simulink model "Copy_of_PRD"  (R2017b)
settings: Solver=FixedStepDiscrete  StartTime=0.0  StopTime=10.0  FixedStep=0.01  RelTol=1e-3  EnableMultiTasking=on
undefined symbols (not defined in the file): CcPRD_MaxPreChrgCnt_numb, CcPRD_PackCurrRat_pct, CcPRD_PreChrgCrntRvsCrntThrd_A, CcPRD_PreChrgCrntRvsDebTi_ms, CcPRD_PreChrgFailWaitTi_s, CcPRD_PreChrgR_ohm, CcPRD_PreChrgShrtDebTi_ms, CcPRD_PreChrgVoltRat_pct, CcPRD_VoltDiff_V, Enum_CTCCtrCtlState, PRD_CONST0_NUMB, PRD_CONST165_NUMB, PRD_CONST60_NUMB, PRD_RUNTIME_MS
libraries: AIWAYS_Powertrain_BMS_lib x17

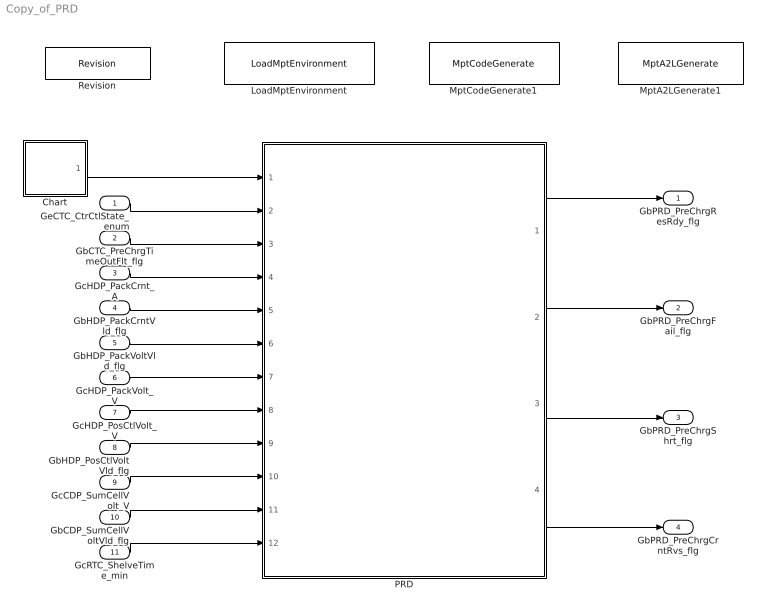
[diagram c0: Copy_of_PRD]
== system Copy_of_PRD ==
  GeCTC_CtrCtlState_enum : Inport
  GbCTC_PreChrgTimeOutFlt_flg : Inport  Port=2
  GcHDP_PackCrnt_A : Inport  Port=3
  GbHDP_PackCrntVld_flg : Inport  Port=4
  GbHDP_PackVoltVld_flg : Inport  Port=5
  GcHDP_PackVolt_V : Inport  Port=6
  GcHDP_PosCtlVolt_V : Inport  Port=7
  GbHDP_PosCtlVoltVld_flg : Inport  Port=8
  GcCDP_SumCellVolt_V : Inport  Port=9
  GbCDP_SumCellVoltVld_flg : Inport  Port=10
  GcRTC_ShelveTime_min : Inport  Port=11
  Chart : Stateflow chart  TreatAsAtomicUnit=on
  LoadMptEnvironment : AIWAYS_Powertrain_BMS_lib/Config/LoadMptEnvironment  ProjectName=Comm  SuppierID=NewPlatformUAES
  MptA2LGenerate1 : AIWAYS_Powertrain_BMS_lib/Config/MptA2LGenerate  SystemSampleTime=-1
  MptCodeGenerate1 : AIWAYS_Powertrain_BMS_lib/Config/MptCodeGenerate  SystemSampleTime=-1
  PRD : Subsystem
  Revision : AIWAYS_Powertrain_BMS_lib/Config/Revision  curVersion='M100C100R101'  newVersion='M100C100R101'
  GbPRD_PreChrgResRdy_flg : Outport
  GbPRD_PreChrgFail_flg : Outport  Port=2
  GbPRD_PreChrgShrt_flg : Outport  Port=3
  GbPRD_PreChrgCrntRvs_flg : Outport  Port=4
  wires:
  GcHDP_PackCrnt_A/1 -> PRD/4(GcHDP_PackCrnt_A)
  GbCTC_PreChrgTimeOutFlt_flg/1 -> PRD/3(GbCTC_PreChrgTimeOutFlt_flg)
  GbHDP_PackCrntVld_flg/1 -> PRD/5(GbHDP_PackCrntVld_flg)
  GeCTC_CtrCtlState_enum/1 -> PRD/2(GeCTC_CtrCtlState_enum)
  GbHDP_PackVoltVld_flg/1 -> PRD/6(GbHDP_PackVoltVld_flg)
  GcHDP_PackVolt_V/1 -> PRD/7(GcHDP_PackVolt_V)
  GcHDP_PosCtlVolt_V/1 -> PRD/8(GcHDP_PosCtlVolt_V)
  GbHDP_PosCtlVoltVld_flg/1 -> PRD/9(GbHDP_PosCtlVoltVld_flg)
  GcCDP_SumCellVolt_V/1 -> PRD/10(GcCDP_SumCellVolt_V)
  GbCDP_SumCellVoltVld_flg/1 -> PRD/11(GbCDP_SumCellVoltVld_flg)
  GcRTC_ShelveTime_min/1 -> PRD/12(GcRTC_ShelveTime_min)
  PRD/1(GbPRD_PreChrgResRdy_flg) -> GbPRD_PreChrgResRdy_flg/1
  PRD/2(GbPRD_PreChrgFail_flg) -> GbPRD_PreChrgFail_flg/1
  PRD/3(GbPRD_PreChrgShrt_flg) -> GbPRD_PreChrgShrt_flg/1
  PRD/4(GbPRD_PreChrgCrntRvs_flg) -> GbPRD_PreChrgCrntRvs_flg/1
  Chart/1(PRD_PreChrgResDiag_10ms()) -> PRD/1(PRD_PreChrgResDiag_10ms)

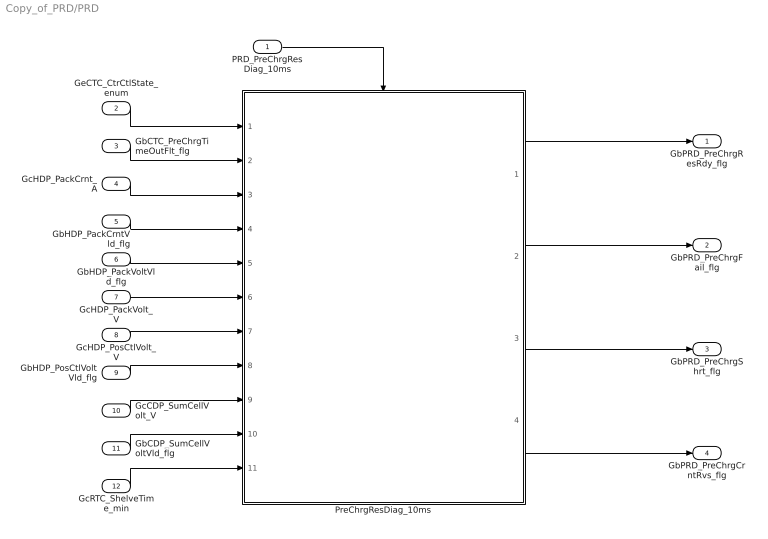
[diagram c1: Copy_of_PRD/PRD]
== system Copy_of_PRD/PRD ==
  PRD_PreChrgResDiag_10ms : Inport
  GeCTC_CtrCtlState_enum : Inport  Port=2
  GbCTC_PreChrgTimeOutFlt_flg : Inport  Port=3
  GcHDP_PackCrnt_A : Inport  Port=4
  GbHDP_PackCrntVld_flg : Inport  Port=5
  GbHDP_PackVoltVld_flg : Inport  Port=6
  GcHDP_PackVolt_V : Inport  Port=7
  GcHDP_PosCtlVolt_V : Inport  Port=8
  GbHDP_PosCtlVoltVld_flg : Inport  Port=9
  GcCDP_SumCellVolt_V : Inport  Port=10
  GbCDP_SumCellVoltVld_flg : Inport  Port=11
  GcRTC_ShelveTime_min : Inport  Port=12
  PreChrgResDiag_10ms : Subsystem
  GbPRD_PreChrgResRdy_flg : Outport
  GbPRD_PreChrgFail_flg : Outport  Port=2
  GbPRD_PreChrgShrt_flg : Outport  Port=3
  GbPRD_PreChrgCrntRvs_flg : Outport  Port=4
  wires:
  GeCTC_CtrCtlState_enum/1 -> PreChrgResDiag_10ms/1(GeCTC_CtrCtlState_enum)
  GbCTC_PreChrgTimeOutFlt_flg/1 -> PreChrgResDiag_10ms/2(GbCTC_PreChrgTimeOutFlt_flg)
  GcHDP_PackCrnt_A/1 -> PreChrgResDiag_10ms/3(GcHDP_PackCrnt_A)
  GbHDP_PackCrntVld_flg/1 -> PreChrgResDiag_10ms/4(GbHDP_PackCrntVld_flg)
  GbHDP_PackVoltVld_flg/1 -> PreChrgResDiag_10ms/5(GbHDP_PackVoltVld_flg)
  GcHDP_PackVolt_V/1 -> PreChrgResDiag_10ms/6(GcHDP_PackVolt_V)
  GcHDP_PosCtlVolt_V/1 -> PreChrgResDiag_10ms/7(GcHDP_PosCtlVolt_V)
  GbHDP_PosCtlVoltVld_flg/1 -> PreChrgResDiag_10ms/8(GbHDP_PosCtlVoltVld_flg)
  GcCDP_SumCellVolt_V/1 -> PreChrgResDiag_10ms/9(GcCDP_SumCellVolt_V)
  GbCDP_SumCellVoltVld_flg/1 -> PreChrgResDiag_10ms/10(GbCDP_SumCellVoltVld_flg)
  GcRTC_ShelveTime_min/1 -> PreChrgResDiag_10ms/11(GcRTC_ShelveTime_min)
  PreChrgResDiag_10ms/1(GbPRD_PreChrgResRdy_flg) -> GbPRD_PreChrgResRdy_flg/1
  PreChrgResDiag_10ms/2(GbPRD_PreChrgFail_flg) -> GbPRD_PreChrgFail_flg/1
  PreChrgResDiag_10ms/3(GbPRD_PreChrgShrt_flg) -> GbPRD_PreChrgShrt_flg/1
  PreChrgResDiag_10ms/4(GbPRD_PreChrgCrntRvs_flg) -> GbPRD_PreChrgCrntRvs_flg/1
  PRD_PreChrgResDiag_10ms/1 -> PreChrgResDiag_10ms/Trigger

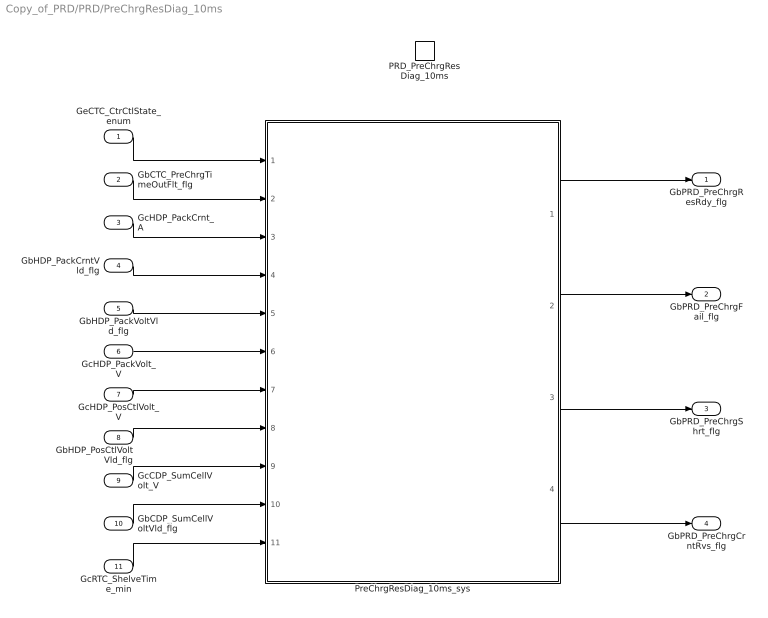
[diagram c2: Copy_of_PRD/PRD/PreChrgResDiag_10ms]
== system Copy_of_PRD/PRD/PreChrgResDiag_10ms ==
  GeCTC_CtrCtlState_enum : Inport
  GbCTC_PreChrgTimeOutFlt_flg : Inport  Port=2
  GcHDP_PackCrnt_A : Inport  Port=3
  GbHDP_PackCrntVld_flg : Inport  Port=4
  GbHDP_PackVoltVld_flg : Inport  Port=5
  GcHDP_PackVolt_V : Inport  Port=6
  GcHDP_PosCtlVolt_V : Inport  Port=7
  GbHDP_PosCtlVoltVld_flg : Inport  Port=8
  GcCDP_SumCellVolt_V : Inport  Port=9
  GbCDP_SumCellVoltVld_flg : Inport  Port=10
  GcRTC_ShelveTime_min : Inport  Port=11
  PRD_PreChrgResDiag_10ms : TriggerPort  TriggerType=function-call  VariantControl=(inherit)
  PreChrgResDiag_10ms_sys : Subsystem
  GbPRD_PreChrgResRdy_flg : Outport
  GbPRD_PreChrgFail_flg : Outport  Port=2
  GbPRD_PreChrgShrt_flg : Outport  Port=3
  GbPRD_PreChrgCrntRvs_flg : Outport  Port=4
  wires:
  PreChrgResDiag_10ms_sys/1(GbPRD_PreChrgResRdy_flg) -> GbPRD_PreChrgResRdy_flg/1
  PreChrgResDiag_10ms_sys/2(GbPRD_PreChrgFail_flg) -> GbPRD_PreChrgFail_flg/1
  PreChrgResDiag_10ms_sys/3(GbPRD_PreChrgShrt_flg) -> GbPRD_PreChrgShrt_flg/1
  PreChrgResDiag_10ms_sys/4(GbPRD_PreChrgCrntRvs_flg) -> GbPRD_PreChrgCrntRvs_flg/1
  GeCTC_CtrCtlState_enum/1 -> PreChrgResDiag_10ms_sys/1(GeCTC_CtrCtlState_enum)
  GbCTC_PreChrgTimeOutFlt_flg/1 -> PreChrgResDiag_10ms_sys/2(GbCTC_PreChrgTimeOutFlt_flg)
  GcHDP_PackCrnt_A/1 -> PreChrgResDiag_10ms_sys/3(GcHDP_PackCrnt_A)
  GbHDP_PackCrntVld_flg/1 -> PreChrgResDiag_10ms_sys/4(GbHDP_PackCrntVld_flg)
  GbHDP_PackVoltVld_flg/1 -> PreChrgResDiag_10ms_sys/5(GbHDP_PackVoltVld_flg)
  GcHDP_PackVolt_V/1 -> PreChrgResDiag_10ms_sys/6(GcHDP_PackVolt_V)
  GcHDP_PosCtlVolt_V/1 -> PreChrgResDiag_10ms_sys/7(GcHDP_PosCtlVolt_V)
  GbHDP_PosCtlVoltVld_flg/1 -> PreChrgResDiag_10ms_sys/8(GbHDP_PosCtlVoltVld_flg)
  GcCDP_SumCellVolt_V/1 -> PreChrgResDiag_10ms_sys/9(GcCDP_SumCellVolt_V)
  GbCDP_SumCellVoltVld_flg/1 -> PreChrgResDiag_10ms_sys/10(GbCDP_SumCellVoltVld_flg)
  GcRTC_ShelveTime_min/1 -> PreChrgResDiag_10ms_sys/11(GcRTC_ShelveTime_min)

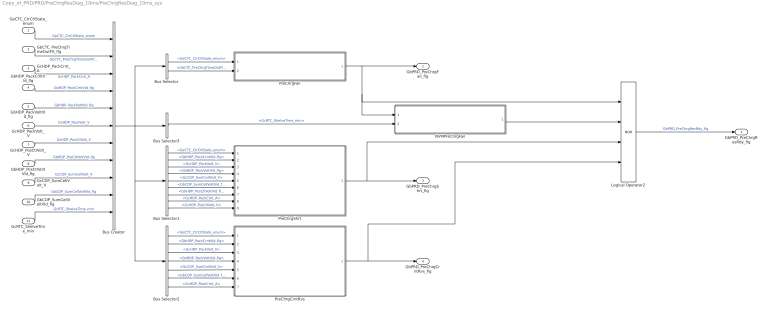
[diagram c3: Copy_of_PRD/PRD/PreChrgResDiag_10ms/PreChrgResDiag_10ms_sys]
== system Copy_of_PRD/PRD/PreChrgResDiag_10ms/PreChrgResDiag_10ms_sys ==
  GeCTC_CtrCtlState_enum : Inport
  GbCTC_PreChrgTimeOutFlt_flg : Inport  Port=2
  GcHDP_PackCrnt_A : Inport  Port=3
  GbHDP_PackCrntVld_flg : Inport  Port=4
  GbHDP_PackVoltVld_flg : Inport  Port=5
  GcHDP_PackVolt_V : Inport  Port=6
  GcHDP_PosCtlVolt_V : Inport  Port=7
  GbHDP_PosCtlVoltVld_flg : Inport  Port=8
  GcCDP_SumCellVolt_V : Inport  Port=9
  GbCDP_SumCellVoltVld_flg : Inport  Port=10
  GcRTC_ShelveTime_min : Inport  Port=11
  Bus Creator : BusCreator  Inputs=11
  Bus Selector : BusSelector  OutputSignals=GeCTC_CtrCtlState_enum,GbCTC_PreChrgTimeOutFlt_flg
  Bus Selector1 : BusSelector  OutputSignals=GeCTC_CtrCtlState_enum,GbHDP_PackCrntVld_flg,GcHDP_PackVolt_V,GbHDP_PackVoltVld_flg,GcCDP_SumCellVolt_V,GbCDP_SumCellVoltVld_flg,GbHDP_PosCtlVoltVld_flg,GcHDP_PackCrnt_A,GcHDP_PosCtlVolt_V
  Bus Selector2 : BusSelector  OutputSignals=GeCTC_CtrCtlState_enum,GbHDP_PackCrntVld_flg,GcHDP_PackVolt_V,GbHDP_PackVoltVld_flg,GcCDP_SumCellVolt_V,GbCDP_SumCellVoltVld_flg,GcHDP_PackCrnt_A
  Bus Selector3 : BusSelector  OutputSignals=GcRTC_ShelveTime_min
  Logical Operator2 : Logic  Operator=NOR  Inputs=4  AllPortsSameDT=off  OutDataTypeStr=boolean
  NVMPreChrgFail : Subsystem
  PreChrgCrntRvs : Subsystem
  PreChrgFail : Subsystem
  PreChrgShrt : Subsystem
  GbPRD_PreChrgResRdy_flg : Outport
  GbPRD_PreChrgFail_flg : Outport  Port=2
  GbPRD_PreChrgShrt_flg : Outport  Port=3
  GbPRD_PreChrgCrntRvs_flg : Outport  Port=4
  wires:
  GbCDP_SumCellVoltVld_flg/1 -> Bus Creator/10  "GbCDP_SumCellVoltVld_flg"
  GbCTC_PreChrgTimeOutFlt_flg/1 -> Bus Creator/2  "GbCTC_PreChrgTimeOutFlt_flg"
  GcCDP_SumCellVolt_V/1 -> Bus Creator/9  "GcCDP_SumCellVolt_V"
  GcHDP_PackCrnt_A/1 -> Bus Creator/3  "GcHDP_PackCrnt_A"
  GcRTC_ShelveTime_min/1 -> Bus Creator/11  "GcRTC_ShelveTime_min"
  GbHDP_PosCtlVoltVld_flg/1 -> Bus Creator/8  "GbHDP_PosCtlVoltVld_flg"
  GeCTC_CtrCtlState_enum/1 -> Bus Creator/1  "GeCTC_CtrCtlState_enum"
  GcHDP_PosCtlVolt_V/1 -> Bus Creator/7  "GcHDP_PosCtlVolt_V"
  GbHDP_PackCrntVld_flg/1 -> Bus Creator/4  "GbHDP_PackCrntVld_flg"
  GcHDP_PackVolt_V/1 -> Bus Creator/6  "GcHDP_PackVolt_V"
  GbHDP_PackVoltVld_flg/1 -> Bus Creator/5  "GbHDP_PackVoltVld_flg"
  Bus Creator/1 -> Bus Selector2/1, Bus Selector1/1, Bus Selector3/1, Bus Selector/1
  Bus Selector/1 -> PreChrgFail/1(GeCTC_CtrCtlState_enum)  "<GeCTC_CtrCtlState_enum>"
  Bus Selector/2 -> PreChrgFail/2(GbCTC_PreChrgTimeOutFlt_flg)  "<GbCTC_PreChrgTimeOutFlt_flg>"
  PreChrgFail/1(GbPRD_PreChrgFail_flg) -> Logical Operator2/1, NVMPreChrgFail/1(GbPRD_PreChrgFail_flg), GbPRD_PreChrgFail_flg/1
  Bus Selector1/2 -> PreChrgShrt/2(GbHDP_PackCrntVld_flg)  "<GbHDP_PackCrntVld_flg>"
  Bus Selector1/1 -> PreChrgShrt/1(GeCTC_CtrCtlState_enum)  "<GeCTC_CtrCtlState_enum>"
  PreChrgShrt/1(GbPRD_PreChrgShrt_flg) -> Logical Operator2/3, GbPRD_PreChrgShrt_flg/1
  Bus Selector1/3 -> PreChrgShrt/3(GcHDP_PackVolt_V)  "<GcHDP_PackVolt_V>"
  Bus Selector1/4 -> PreChrgShrt/4(GbHDP_PackVoltVld_flg)  "<GbHDP_PackVoltVld_flg>"
  Bus Selector1/5 -> PreChrgShrt/5(GcCDP_SumCellVolt_V)  "<GcCDP_SumCellVolt_V>"
  Bus Selector1/6 -> PreChrgShrt/6(GbCDP_SumCellVoltVld_flg)  "<GbCDP_SumCellVoltVld_flg>"
  Bus Selector1/7 -> PreChrgShrt/7(GbHDP_PosCtlVoltVld_flg)  "<GbHDP_PosCtlVoltVld_flg>"
  Bus Selector1/8 -> PreChrgShrt/8(GcHDP_PackCrnt_A)  "<GcHDP_PackCrnt_A>"
  Bus Selector1/9 -> PreChrgShrt/9(GcHDP_PosCtlVolt_V)  "<GcHDP_PosCtlVolt_V>"
  Bus Selector2/1 -> PreChrgCrntRvs/1(GeCTC_CtrCtlState_enum)  "<GeCTC_CtrCtlState_enum>"
  Bus Selector2/2 -> PreChrgCrntRvs/2(GbHDP_PackCrntVld_flg)  "<GbHDP_PackCrntVld_flg>"
  Bus Selector2/3 -> PreChrgCrntRvs/3(GcHDP_PackVolt_V)  "<GcHDP_PackVolt_V>"
  Bus Selector2/4 -> PreChrgCrntRvs/4(GbHDP_PackVoltVld_flg)  "<GbHDP_PackVoltVld_flg>"
  Bus Selector2/5 -> PreChrgCrntRvs/5(GcCDP_SumCellVolt_V)  "<GcCDP_SumCellVolt_V>"
  Bus Selector2/6 -> PreChrgCrntRvs/6(GbCDP_SumCellVoltVld_flg)  "<GbCDP_SumCellVoltVld_flg>"
  Bus Selector2/7 -> PreChrgCrntRvs/7(GcHDP_PackCrnt_A)  "<GcHDP_PackCrnt_A>"
  PreChrgCrntRvs/1(GbPRD_PreChrgCrntRvs_flg) -> Logical Operator2/4, GbPRD_PreChrgCrntRvs_flg/1
  Bus Selector3/1 -> NVMPreChrgFail/2(GcRTC_ShelveTime_min)  "<GcRTC_ShelveTime_min>"
  Logical Operator2/1 -> GbPRD_PreChrgResRdy_flg/1  "GbPRD_PreChrgResRdy_flg"
  NVMPreChrgFail/1(LbPRD_NVMPreChrgFail_flg) -> Logical Operator2/2

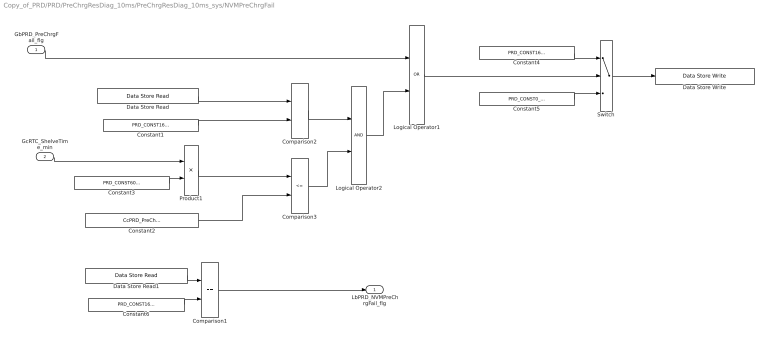
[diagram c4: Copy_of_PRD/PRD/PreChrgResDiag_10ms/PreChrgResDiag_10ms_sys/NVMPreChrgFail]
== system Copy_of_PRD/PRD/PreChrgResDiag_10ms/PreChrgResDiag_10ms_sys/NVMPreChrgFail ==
  GbPRD_PreChrgFail_flg : Inport
  GcRTC_ShelveTime_min : Inport  Port=2
  Comparison1 : RelationalOperator  Operator===  OutDataTypeStr=boolean
  Comparison2 : RelationalOperator  Operator===  OutDataTypeStr=boolean
  Comparison3 : RelationalOperator  Operator=<=  OutDataTypeStr=boolean
  Constant1 : Constant  Value=PRD_CONST165_NUMB
  Constant2 : Constant  Value=CcPRD_PreChrgFailWaitTi_s
  Constant3 : Constant  Value=PRD_CONST60_NUMB
  Constant4 : Constant  Value=PRD_CONST165_NUMB
  Constant5 : Constant  Value=PRD_CONST0_NUMB
  Constant6 : Constant  Value=PRD_CONST165_NUMB
  Data Store Read : AIWAYS_Powertrain_BMS_lib/Signals/Data Store Read  Priority=0  DSR=EcNVM_NVMPreChrgFail_numb
  Data Store Read1 : AIWAYS_Powertrain_BMS_lib/Signals/Data Store Read  Priority=0  DSR=EcNVM_NVMPreChrgFail_numb
  Data Store Write : AIWAYS_Powertrain_BMS_lib/Signals/Data Store Write  DSW=EcNVM_NVMPreChrgFail_numb
  Logical Operator1 : Logic  Operator=OR  AllPortsSameDT=off  OutDataTypeStr=boolean
  Logical Operator2 : Logic  AllPortsSameDT=off  OutDataTypeStr=boolean
  Product1 : Product  Inputs=**  OutDataTypeStr=uint32
  Switch : Switch  Criteria=u2 ~= 0  Threshold=1  RndMeth=Zero
  LbPRD_NVMPreChrgFail_flg : Outport
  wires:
  Data Store Read/1 -> Comparison2/1
  Constant1/1 -> Comparison2/2
  Comparison2/1 -> Logical Operator2/1
  Comparison3/1 -> Logical Operator2/2
  Product1/1 -> Comparison3/1
  GcRTC_ShelveTime_min/1 -> Product1/1
  Constant3/1 -> Product1/2
  Constant2/1 -> Comparison3/2
  GbPRD_PreChrgFail_flg/1 -> Logical Operator1/1
  Logical Operator2/1 -> Logical Operator1/2
  Logical Operator1/1 -> Switch/2
  Switch/1 -> Data Store Write/1
  Constant4/1 -> Switch/1
  Constant5/1 -> Switch/3
  Constant6/1 -> Comparison1/2
  Data Store Read1/1 -> Comparison1/1
  Comparison1/1 -> LbPRD_NVMPreChrgFail_flg/1

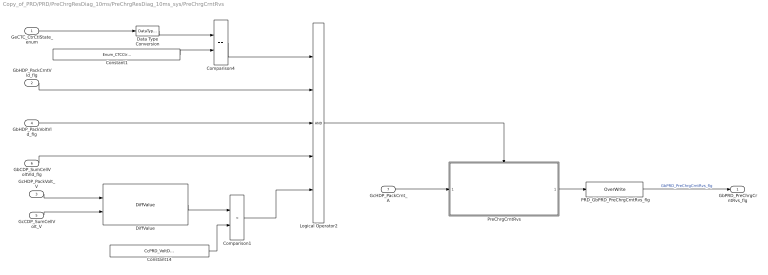
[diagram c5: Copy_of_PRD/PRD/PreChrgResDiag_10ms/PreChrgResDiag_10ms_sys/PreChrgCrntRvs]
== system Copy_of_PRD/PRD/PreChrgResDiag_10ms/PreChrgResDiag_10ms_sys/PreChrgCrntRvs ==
  GeCTC_CtrCtlState_enum : Inport
  GbHDP_PackCrntVld_flg : Inport  Port=2
  GcHDP_PackVolt_V : Inport  Port=3
  GbHDP_PackVoltVld_flg : Inport  Port=4
  GcCDP_SumCellVolt_V : Inport  Port=5
  GbCDP_SumCellVoltVld_flg : Inport  Port=6
  GcHDP_PackCrnt_A : Inport  Port=7
  Comparison1 : RelationalOperator  Operator=<  OutDataTypeStr=boolean
  Comparison4 : RelationalOperator  Operator===  OutDataTypeStr=boolean
  Constant1 : Constant  Value=Enum_CTCCtrCtlState.Enum_CTCCtrCtlState_Connect
  Constant14 : Constant  Value=CcPRD_VoltDiff_V
  Data Type Conversion : DataTypeConversion
  DiffValue : AIWAYS_Powertrain_BMS_lib/Mathematical Functions/DiffValue
  Logical Operator2 : Logic  Inputs=5  AllPortsSameDT=off  OutDataTypeStr=boolean
  PRD_GbPRD_PreChrgCrntRvs_flg : AIWAYS_Powertrain_BMS_lib/Signals/OverWrite  OverWrite_Value=CbPRD_PreChrgCrntRvsOvr_flg  OverWrite_flag=CbPRD_PreChrgCrntRvsOvrSwt_flg
  PreChrgCrntRvs : Subsystem
  GbPRD_PreChrgCrntRvs_flg : Outport
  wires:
  Constant1/1 -> Comparison4/2
  Data Type Conversion/1 -> Comparison4/1
  GeCTC_CtrCtlState_enum/1 -> Data Type Conversion/1
  Comparison4/1 -> Logical Operator2/1
  GcCDP_SumCellVolt_V/1 -> DiffValue/2
  Constant14/1 -> Comparison1/2
  DiffValue/1 -> Comparison1/1
  Logical Operator2/1 -> PreChrgCrntRvs/Enable
  PreChrgCrntRvs/1(GbPRD_PreChrgCrntRvs_flg) -> PRD_GbPRD_PreChrgCrntRvs_flg/1
  GcHDP_PackVolt_V/1 -> DiffValue/1
  GcHDP_PackCrnt_A/1 -> PreChrgCrntRvs/1(GcHDP_PackCrnt_A)
  GbHDP_PackCrntVld_flg/1 -> Logical Operator2/2
  GbHDP_PackVoltVld_flg/1 -> Logical Operator2/3
  GbCDP_SumCellVoltVld_flg/1 -> Logical Operator2/4
  Comparison1/1 -> Logical Operator2/5
  PRD_GbPRD_PreChrgCrntRvs_flg/1 -> GbPRD_PreChrgCrntRvs_flg/1  "GbPRD_PreChrgCrntRvs_flg"

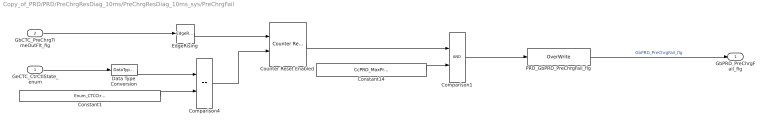
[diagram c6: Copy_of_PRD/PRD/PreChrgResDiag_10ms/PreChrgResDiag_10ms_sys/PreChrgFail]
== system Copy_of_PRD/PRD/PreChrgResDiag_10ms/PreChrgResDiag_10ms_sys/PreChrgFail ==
  GeCTC_CtrCtlState_enum : Inport
  GbCTC_PreChrgTimeOutFlt_flg : Inport  Port=2
  Comparison1 : RelationalOperator  OutDataTypeStr=boolean
  Comparison4 : RelationalOperator  Operator===  OutDataTypeStr=boolean
  Constant1 : Constant  Value=Enum_CTCCtrCtlState.Enum_CTCCtrCtlState_Online
  Constant14 : Constant  Value=CcPRD_MaxPreChrgCnt_numb
  "Counter Reset Enabled " : AIWAYS_Powertrain_BMS_lib/Counters & Timers/Counter Reset  Enabled 
  Data Type Conversion : DataTypeConversion
  EdgeRising : AIWAYS_Powertrain_BMS_lib/Logical Operators/EdgeRising
  PRD_GbPRD_PreChrgFail_flg : AIWAYS_Powertrain_BMS_lib/Signals/OverWrite  OverWrite_Value=CbPRD_PreChrgFailOvr_flg  OverWrite_flag=CbPRD_PreChrgFailOvrSwt_flg
  GbPRD_PreChrgFail_flg : Outport
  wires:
  EdgeRising/1 -> "Counter Reset Enabled "/1
  GbCTC_PreChrgTimeOutFlt_flg/1 -> EdgeRising/1
  GeCTC_CtrCtlState_enum/1 -> Data Type Conversion/1
  Data Type Conversion/1 -> Comparison4/1
  Comparison4/1 -> "Counter Reset Enabled "/2
  Comparison1/1 -> PRD_GbPRD_PreChrgFail_flg/1
  "Counter Reset Enabled "/1 -> Comparison1/1
  Constant1/1 -> Comparison4/2
  Constant14/1 -> Comparison1/2
  PRD_GbPRD_PreChrgFail_flg/1 -> GbPRD_PreChrgFail_flg/1  "GbPRD_PreChrgFail_flg"

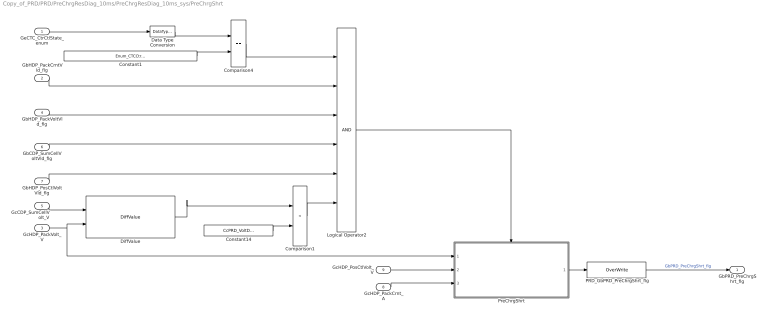
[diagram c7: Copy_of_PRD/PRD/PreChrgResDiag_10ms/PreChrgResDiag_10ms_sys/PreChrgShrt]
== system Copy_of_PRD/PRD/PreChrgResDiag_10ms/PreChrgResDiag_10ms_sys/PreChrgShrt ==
  GeCTC_CtrCtlState_enum : Inport
  GbHDP_PackCrntVld_flg : Inport  Port=2
  GcHDP_PackVolt_V : Inport  Port=3
  GbHDP_PackVoltVld_flg : Inport  Port=4
  GcCDP_SumCellVolt_V : Inport  Port=5
  GbCDP_SumCellVoltVld_flg : Inport  Port=6
  GbHDP_PosCtlVoltVld_flg : Inport  Port=7
  GcHDP_PackCrnt_A : Inport  Port=8
  GcHDP_PosCtlVolt_V : Inport  Port=9
  Comparison1 : RelationalOperator  Operator=<  OutDataTypeStr=boolean
  Comparison4 : RelationalOperator  Operator===  OutDataTypeStr=boolean
  Constant1 : Constant  Value=Enum_CTCCtrCtlState.Enum_CTCCtrCtlState_Connect
  Constant14 : Constant  Value=CcPRD_VoltDiff_V
  Data Type Conversion : DataTypeConversion
  DiffValue : AIWAYS_Powertrain_BMS_lib/Mathematical Functions/DiffValue
  Logical Operator2 : Logic  Inputs=6  AllPortsSameDT=off  OutDataTypeStr=boolean
  PRD_GbPRD_PreChrgShrt_flg : AIWAYS_Powertrain_BMS_lib/Signals/OverWrite  OverWrite_Value=CbPRD_PreChrgShrtOvr_flg  OverWrite_flag=CbPRD_PreChrgShrtOvrSwt_flg
  PreChrgShrt : Subsystem
  GbPRD_PreChrgShrt_flg : Outport
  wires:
  Constant1/1 -> Comparison4/2
  Data Type Conversion/1 -> Comparison4/1
  GeCTC_CtrCtlState_enum/1 -> Data Type Conversion/1
  Comparison4/1 -> Logical Operator2/1
  GbHDP_PackCrntVld_flg/1 -> Logical Operator2/2
  GbHDP_PackVoltVld_flg/1 -> Logical Operator2/3
  GbCDP_SumCellVoltVld_flg/1 -> Logical Operator2/4
  GbHDP_PosCtlVoltVld_flg/1 -> Logical Operator2/5
  Constant14/1 -> Comparison1/2
  DiffValue/1 -> Comparison1/1
  Comparison1/1 -> Logical Operator2/6
  Logical Operator2/1 -> PreChrgShrt/Enable
  PreChrgShrt/1(GbPRD_PreChrgShrt_flg) -> PRD_GbPRD_PreChrgShrt_flg/1
  GcHDP_PackCrnt_A/1 -> PreChrgShrt/3(GcHDP_PackCrnt_A)
  GcHDP_PosCtlVolt_V/1 -> PreChrgShrt/2(GcHDP_PosCtlVolt_V)
  PRD_GbPRD_PreChrgShrt_flg/1 -> GbPRD_PreChrgShrt_flg/1  "GbPRD_PreChrgShrt_flg"
  GcCDP_SumCellVolt_V/1 -> DiffValue/1
  GcHDP_PackVolt_V/1 -> PreChrgShrt/1(GcHDP_PackVolt_V), DiffValue/2

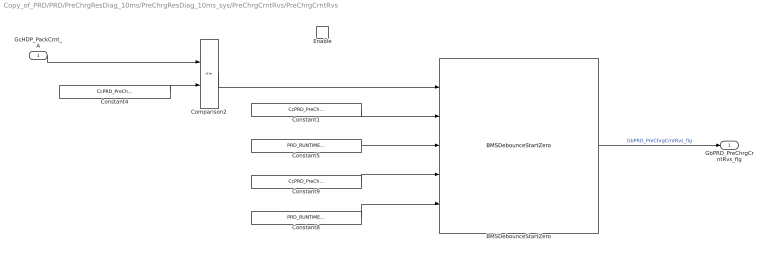
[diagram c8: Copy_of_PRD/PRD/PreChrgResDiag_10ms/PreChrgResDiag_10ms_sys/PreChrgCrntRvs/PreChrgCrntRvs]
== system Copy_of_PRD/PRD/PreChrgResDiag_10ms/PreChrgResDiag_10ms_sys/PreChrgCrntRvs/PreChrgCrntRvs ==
  GcHDP_PackCrnt_A : Inport
  Enable : EnablePort
  BMSDebounceStartZero : AIWAYS_Powertrain_BMS_lib/Debounce & Delay/BMSDebounceStartZero
  Comparison2 : RelationalOperator  Operator=<=  OutDataTypeStr=boolean
  Constant1 : Constant  Value=CcPRD_PreChrgCrntRvsDebTi_ms
  Constant4 : Constant  Value=CcPRD_PreChrgCrntRvsCrntThrd_A
  Constant5 : Constant  Value=PRD_RUNTIME_MS
  Constant8 : Constant  Value=PRD_RUNTIME_MS
  Constant9 : Constant  Value=CcPRD_PreChrgCrntRvsDebTi_ms
  GbPRD_PreChrgCrntRvs_flg : Outport
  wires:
  Constant5/1 -> BMSDebounceStartZero/3
  Constant8/1 -> BMSDebounceStartZero/5
  Constant9/1 -> BMSDebounceStartZero/4
  Constant1/1 -> BMSDebounceStartZero/2
  BMSDebounceStartZero/1 -> GbPRD_PreChrgCrntRvs_flg/1  "GbPRD_PreChrgCrntRvs_flg"
  Constant4/1 -> Comparison2/2
  GcHDP_PackCrnt_A/1 -> Comparison2/1
  Comparison2/1 -> BMSDebounceStartZero/1

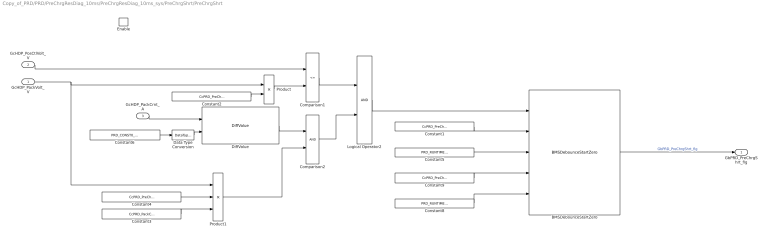
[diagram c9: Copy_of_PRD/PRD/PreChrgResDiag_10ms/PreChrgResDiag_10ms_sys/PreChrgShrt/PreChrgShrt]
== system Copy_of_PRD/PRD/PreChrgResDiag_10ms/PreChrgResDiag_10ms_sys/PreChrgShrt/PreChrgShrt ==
  GcHDP_PackVolt_V : Inport
  GcHDP_PosCtlVolt_V : Inport  Port=2
  GcHDP_PackCrnt_A : Inport  Port=3
  Enable : EnablePort
  BMSDebounceStartZero : AIWAYS_Powertrain_BMS_lib/Debounce & Delay/BMSDebounceStartZero
  Comparison1 : RelationalOperator  Operator=<=  OutDataTypeStr=boolean
  Comparison2 : RelationalOperator  OutDataTypeStr=boolean
  Constant1 : Constant  Value=CcPRD_PreChrgShrtDebTi_ms
  Constant2 : Constant  Value=CcPRD_PreChrgVoltRat_pct
  Constant3 : Constant  Value=CcPRD_PackCurrRat_pct
  Constant4 : Constant  Value=CcPRD_PreChrgR_ohm
  Constant5 : Constant  Value=PRD_RUNTIME_MS
  Constant6 : Constant  Value=PRD_CONST0_NUMB
  Constant8 : Constant  Value=PRD_RUNTIME_MS
  Constant9 : Constant  Value=CcPRD_PreChrgShrtDebTi_ms
  Data Type Conversion : DataTypeConversion  OutDataTypeStr=single
  DiffValue : AIWAYS_Powertrain_BMS_lib/Mathematical Functions/DiffValue
  Logical Operator2 : Logic  AllPortsSameDT=off  OutDataTypeStr=boolean
  Product : Product
  Product1 : Product  Inputs=*/*
  GbPRD_PreChrgShrt_flg : Outport
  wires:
  Constant5/1 -> BMSDebounceStartZero/3
  Constant8/1 -> BMSDebounceStartZero/5
  Constant9/1 -> BMSDebounceStartZero/4
  Constant1/1 -> BMSDebounceStartZero/2
  BMSDebounceStartZero/1 -> GbPRD_PreChrgShrt_flg/1  "GbPRD_PreChrgShrt_flg"
  GcHDP_PosCtlVolt_V/1 -> Comparison1/1
  Product/1 -> Comparison1/2
  GcHDP_PackVolt_V/1 -> Product/1, Product1/1
  Constant2/1 -> Product/2
  GcHDP_PackCrnt_A/1 -> DiffValue/1
  Constant3/1 -> Product1/3
  Constant4/1 -> Product1/2
  DiffValue/1 -> Comparison2/1
  Product1/1 -> Comparison2/2
  Comparison1/1 -> Logical Operator2/1
  Comparison2/1 -> Logical Operator2/2
  Logical Operator2/1 -> BMSDebounceStartZero/1
  Data Type Conversion/1 -> DiffValue/2
  Constant6/1 -> Data Type Conversion/1

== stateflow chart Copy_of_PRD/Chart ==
  (default) -> (junction 1)
  (junction 1) -> (junction 3) : {PRD_PreChrgResDiag_10ms;}
  events: output FUNCTION_CALL_EVENT
